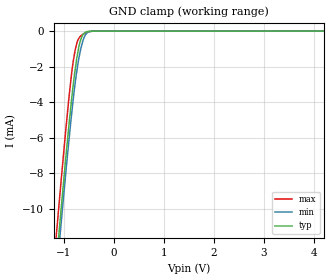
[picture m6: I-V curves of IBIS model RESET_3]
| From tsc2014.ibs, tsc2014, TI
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|   3.0V RESET Model
[Model] RESET_3
Model_type Input
Vinl = 0.9
Vinh = 2.1
|   typ   min   max
C_comp   2.0467170e-12   1.9248300e-12   2.1797870e-12
|Where nom PVT is NOM Process, 3V,27C
|   Fast PVT is Strong Process, 3.45V, -40C
|   Slow PVT is Weak Process, 2.65V, 85C
[Model Spec]
Vinl   0.9   0.795   1.035
Vinh   2.1   1.855   2.415
| VINL 0.3 DVDD, VINH 0.7 DVDD
[Voltage Range]   3   2.65   3.45
[Temperature Range]   27   85   -40
[Power Clamp Reference]   3   2.65   3.45
[GND Clamp Reference]   0   0   0
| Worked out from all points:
|   GND clamp passes 1 mA (typ) near -0.71 V on its own axis
[GND Clamp]
|   Voltage   I(typ)   I(min)   I(max)
-3V       -76.36mA   -75.99mA   -75.93mA
-1.144V   -12.89mA   -13.67mA   -11.3mA
-1.095V   -11.33mA   -12.12mA   -9.736mA
-1.069V   -10.48mA   -11.29mA   -8.885mA
-1.057V   -10.11mA   -10.92mA   -8.513mA
-902.6mV  -5.435mA   -6.29mA    -3.884mA
-809.4mV  -2.977mA   -3.779mA   -1.661mA
-735mV    -1.437mA   -2.158mA   -634.2uA
-696.4mV  -858.6uA   -1.495mA   -397.3uA
-578.1mV  -84.31uA   -266.3uA   -119.7uA
-408.4mV  -2.578uA   -2.581uA   -2.635uA
6V        0A         0A         0A
[POWER Clamp]
|   SCR cell used for ESD function. Effects occurr above VDD x 2
|   Voltage   I(typ)   I(min)   I(max)
-3V       0A         0A         0A
0V        0A         0A         0A
6V        0A         0A         0A
